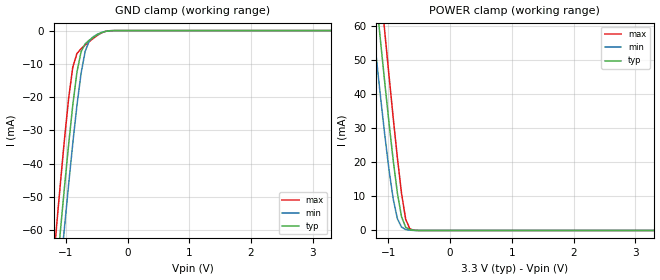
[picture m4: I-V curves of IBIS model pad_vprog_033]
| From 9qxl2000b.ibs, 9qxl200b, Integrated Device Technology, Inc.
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|   Model pad_vprog_033
[Model] pad_vprog_033
Model_type Input
Vinl =   0.3000V
Vinh =   0.5000V
Polarity   Non-Inverting
C_comp   1.077pF   1.044pF   1.096pF
C_comp_pullup   82.464fF   75.746fF   85.392fF
[Temperature Range]   65.000   0.125k   -10.000
[Voltage Range]   3.300V   3.135V   3.465V
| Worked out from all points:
|   GND clamp passes 1 mA (typ) near -0.46 V on its own axis
|   POWER clamp passes 1 mA (typ) near -0.72 V on its own axis
[GND_clamp]
|Voltage   I(typ)   I(min)   I(max)
-3.3V     -550.4mA   -550.5mA   -551mA
-1.156V   -74mA      -85.96mA   -59.97mA
-1.089V   -60.3mA    -72.4mA    -45.95mA
-1.022V   -46.96mA   -59.12mA   -32.54mA
-955mV    -34.18mA   -46.22mA   -20.34mA
-888mV    -22.4mA    -33.91mA   -11.02mA
-821mV    -12.55mA   -22.55mA   -6.911mA
-754mV    -6.375mA   -12.89mA   -5.468mA
-687mV    -3.969mA   -6.201mA   -4.351mA
-620mV    -2.864mA   -3.069mA   -3.292mA
-486mV    -1.239mA   -1.074mA   -1.393mA
3.3V      0A         0A         0A
[POWER_clamp]
|Voltage   I(typ)   I(min)   I(max)
-3.3V     476mA      447.8mA    505.4mA
-1.256V   79.07mA    61.22mA    96.1mA
-1.189V   66.73mA    49.58mA    83.12mA
-1.122V   54.58mA    38.27mA    70.25mA
-1.055V   42.7mA     27.48mA    57.53mA
-921mV    20.46mA    9.151mA    32.87mA
-854mV    10.96mA    3.45mA     21.3mA
-787mV    4.033mA    997.8uA    10.91mA
-720mV    969.8uA    297.5uA    3.305mA
-653mV    231.9uA    81.06uA    522.6uA
-519mV    6.233uA    2.7uA      7.095uA
3.3V      0A         0A         302.8pA
